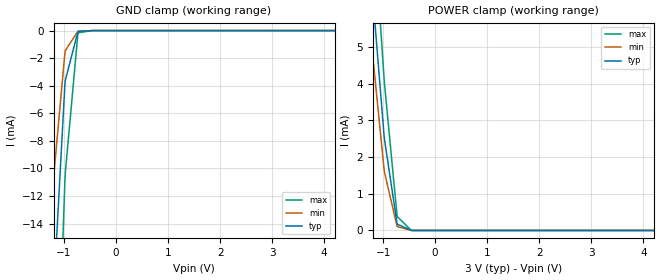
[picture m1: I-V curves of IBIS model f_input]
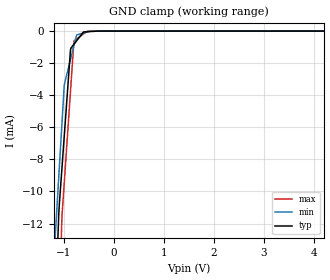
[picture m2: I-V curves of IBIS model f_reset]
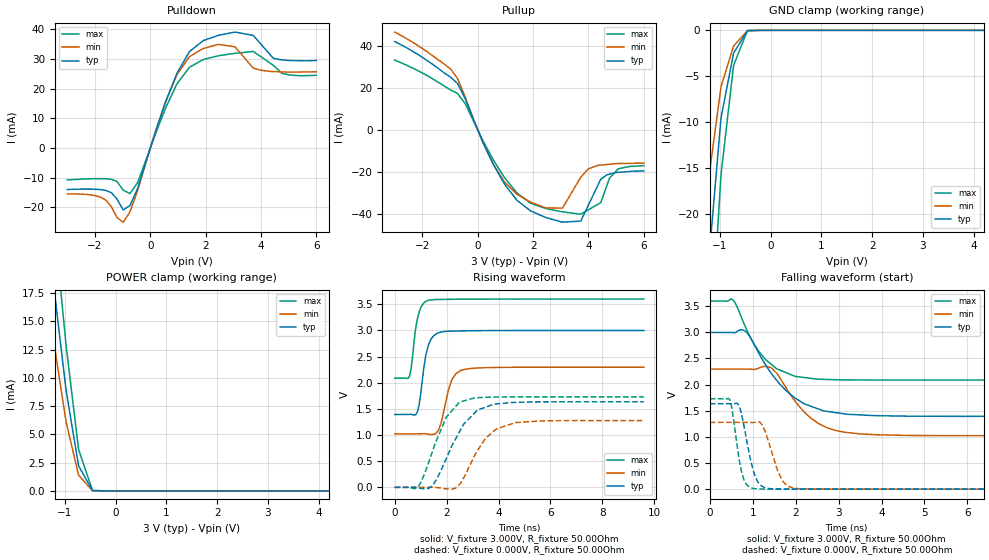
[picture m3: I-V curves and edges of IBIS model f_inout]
[IBIS Ver]   3.2
[File Name]   rc_p33_30v_128m_b.ibs
[File Rev]   1.01
[Date]   8/21/2009
[Source]   From silicon level SPICE model at Numonyx B.V.
[Notes]   The following information corresponds to the
   Redcliff 65nm P33 128Mb chip with EZBGA package.
[Disclaimer]   This information is for modeling purposes only and is not
   guaranteed.Numonyx B.V. is not responsible for any problem
   this model may cause to customers.
[Copyright]   Copyright 2009, Numonyx B.V., All Rights Reserved.
[Component]   P33_30V_128M_EZBGA
[Manufacturer]  Numonyx B.V.
[Package]
|   typ   min   max
R_pkg   0.33Ohm   0.16Ohm   0.50Ohm
L_pkg   6.77nH   3.42nH   10.12nH
C_pkg   1.25pF   0.27pF   2.23pF
[PIN]   signal_name   model_name   R_pin   L_pin   C_pin
A1   A0   f_input   0.28   5.77nH   0.65pF
A2   A5   f_input   0.36   7.41nH   0.92pF
A3   A7   f_input   0.20   4.23nH   0.40pF
A4   NC   NC
A5   A12   f_input   0.16   3.42nH   0.27pF
A6   VCC   POWER
A7   A17   f_input   0.26   5.74nH   0.67pF
A8   A21   f_input   0.33   7.38nH   0.83pF
B1   A1   f_input   0.27   5.51nH   0.60pF
B2   VSS   GND
B3   A8   f_input   0.35   7.25nH   0.89pF
B4   CE#   f_input   0.43   8.13nH   1.28pF
B5   A13   f_input   0.23   4.66nH   0.46pF
B6   NC   NC
B7   A18   f_input   0.26   5.62nH   0.64pF
B8   NC   NC
C1   A2   f_input   0.29   5.77nH   0.64pF
C2   A6   f_input   0.29   5.73nH   0.64pF
C3   A9   f_input   0.35   7.03nH   0.85pF
C4   A11   f_input   0.34   6.86nH   0.82pF
C5   A14   f_input   0.27   5.44nH   0.59pF
C6   WP#   f_input   0.27   5.44nH   0.59pF
C7   A19   f_input   0.41   8.27nH   1.06pF
C8   A20   f_input   0.33   6.76nH   0.81pF
D1   A3   f_input   0.30   6.07nH   0.69pF
D2   A4   f_input   0.28   5.47nH   0.59pF
D3   A10   f_input   0.37   7.50nH   0.93pF
D4   RST#   f_reset   0.32   6.25nH   0.83pF
D5   VCCQ   POWER
D6   VCCQ   POWER
D7   A15   f_input   0.25   4.83nH   0.48pF
D8   A16   f_input   0.29   5.71nH   0.62pF
E1   D8   f_inout   0.28   6.28nH   0.82pF
E2   D1   f_inout   0.26   5.20nH   0.63pF
E3   D9   f_inout   0.25   4.92nH   0.56pF
E4   D3   f_inout   0.25   4.98nH   0.58pF
E5   D4   f_inout   0.30   5.87nH   0.65pF
E6   CLK   f_input   0.29   5.72nH   0.73pF
E7   D15   f_inout   0.27   5.36nH   0.56pF
E8   NC   NC
F1   NC   NC
F2   D0   f_inout   0.21   4.33nH   0.46pF
F3   D10   f_inout   0.23   4.69nH   0.55pF
F4   D11   f_inout   0.23   4.60nH   0.52pF
F5   D12   f_inout   0.20   4.02nH   0.43pF
F6   ADV#   f_input   0.25   4.85nH   0.49pF
F7   WAIT   f_inout   0.24   4.71nH   0.53pF
F8   OE#   f_input   0.42   9.70nH   2.23pF
G1   A22   f_input   0.47   10.12nH   1.28pF
G2   NC   NC
G3   D2   f_inout   0.22   4.43nH   0.42pF
G4   VCCQ   POWER
G5   D5   f_inout   0.17   3.51nH   0.35pF
G6   D6   f_inout   0.18   3.76nH   0.40pF
G7   D14   f_inout   0.22   4.44nH   0.42pF
G8   WE#   f_input   0.50   9.96nH   1.33pF
H1   NC   NC
H2   VSSQ   GND
H3   VCC   POWER
H4   VSS   GND
H5   D13   f_inout   0.21   4.31nH   0.41pF
H6   VSSQ   GND
H7   D7   f_inout   0.23   4.67nH   0.46pF
H8   NC   NC
| Models and submodels in the file (3): f_input (Input), f_reset (Input), f_inout (I/O)
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[Model]   f_input
Model_type   Input
Vinl = 0.400V
Vinh = 2.600V
|   typ   min   max
C_comp   6.000pF   2.000pF   7.000pF
[Voltage Range]   3.000V   2.300V   3.600V
[Temperature Range]   25.0   85.0   -40.0
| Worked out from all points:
|   GND clamp passes 1 mA (typ) near -0.79 V on its own axis
|   POWER clamp passes 1 mA (typ) near -0.82 V on its own axis
[GND Clamp]
|   Voltage   I(typ)   I(min)   I(max)
-3V       -214.2mA   -171.1mA   -282mA
-1.398V   -38.01mA   -24.9mA    -60.4mA
-1.209V   -20.02mA   -11.33mA   -36.27mA
-1.2V     -19.19mA   -10.72mA   -35.15mA
-984mV    -4.085mA   -1.721mA   -11.16mA
-975mV    -3.631mA   -1.46mA    -10.38mA
-732mV    -88.55uA   -49.57uA   -226.8uA
-723mV    -64.96uA   -39.8uA    -159.9uA
-453mV    -377.4nA   -554.6nA   -216.8nA
6V        0A         0A         0A
[POWER Clamp]
|   Voltage   I(typ)   I(min)   I(max)
-3V       44.58mA    39.22mA    51.64mA
-1.299V   8.339mA    6.46mA     11.02mA
-1.209V   6.572mA    4.919mA    8.979mA
-1.2V     6.398mA    4.769mA    8.776mA
-984mV    2.624mA    1.697mA    4.188mA
-975mV    2.493mA    1.595mA    4.017mA
-732mV    187.3uA    115.4uA    401uA
-723mV    168.4uA    103.4uA    368.4uA
-453mV    1.105uA    1.525uA    700.3nA
6V        0A         0A         0A
[Model]   f_reset
Model_type   Input
Vinl = 0.400V
Vinh = 2.600V
|   typ   min   max
C_comp   6.000pF   2.000pF   7.000pF
[Voltage Range]   3.000V   2.300V   3.600V
[Temperature Range]   25.0   85.0   -40.0
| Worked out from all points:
|   GND clamp passes 1 mA (typ) near -0.84 V on its own axis
[GND Clamp]
|   Voltage   I(typ)   I(min)   I(max)
-3V       -205.4mA   -173mA     -256.3mA
-1.209V   -20.5mA    -14.72mA   -29.6mA
-1.101V   -11.42mA   -9.082mA   -18.23mA
-1.047V   -8.959mA   -6.264mA   -12.54mA
-1.038V   -8.571mA   -5.795mA   -11.6mA
-993mV    -6.627mA   -3.447mA   -9.54mA
-867mV    -1.187mA   -1.777mA   -3.783mA
-795mV    -811.6uA   -873.4uA   -609.4uA
-741mV    -594.7uA   -238.1uA   -486.6uA
-606mV    -54.38uA   -121.6uA   -179.4uA
-318mV    -41.02nA   -2.805uA   -2.579uA
6V        0A         0A         0A
[POWER Clamp]
|   Voltage   I(typ)   I(min)   I(max)
-3V       0A         0A         0A
0V        0A         0A         0A
2.301V    0A         0A         0A
3.003V    0A         0A         0A
3.597V    0A         0A         0A
6V        0A         0A         0A
|Note: Typical Pullup/Pulldown I-V drives the most current due to
|silicon process output compensation setting.
[Model]   f_inout
Model_type   I/O
Vinl = 0.400V
Vinh = 2.600V
Vmeas = 1.500V
Vref = 1.500V
Cref = 30.0pF
|   typ   min   max
C_comp   4.000pF   2.000pF   5.000pF
[Voltage Range]   3.000V   2.300V   3.600V
[Temperature Range]   25.0   85.0   -40.0
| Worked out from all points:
|   slope of the pulldown table from 0 to 0.45 V, typ, clamps not added: 35.3 ohm
|   slope of the pullup table from 0 to 0.45 V, typ, clamps not added: 33.6 ohm
|   falling waveform, V_fixture 3.000V, R_fixture 50.00Ohm: 20-80 % time 950ps typ, 795ps min, 698ps max; typ from 3 V to 1.39 V
|   rising waveform, V_fixture 3.000V, R_fixture 50.00Ohm: 20-80 % time 294ps typ, 376ps min, 254ps max; typ from 1.39 V to 3 V
|   rising waveform, V_fixture 0.000V, R_fixture 50.00Ohm: 20-80 % time 1.07ns typ, 959ps min, 850ps max; typ from 0.001 V to 1.64 V
|   falling waveform, V_fixture 0.000V, R_fixture 50.00Ohm: 20-80 % time 252ps typ, 311ps min, 193ps max; typ from 1.64 V to 0.001 V
[Pulldown]
|   Voltage   I(typ)   I(min)   I(max)
-3V       -13.95mA   -15.43mA   -10.69mA
-1.749V   -14.03mA   -16.72mA   -10.29mA
-975mV    -20.83mA   -24.95mA   -14.15mA
-732mV    -19.35mA   -21.46mA   -15.33mA
-453mV    -13.45mA   -14.2mA    -11.51mA
186mV     5.442mA    5.555mA    4.728mA
960mV     25.11mA    24.64mA    21.55mA
1.914V    36.21mA    33.56mA    29.84mA
3.057V    39.08mA    34.14mA    31.92mA
3.723V    37.95mA    26.93mA    32.57mA
4.452V    30.24mA    25.78mA    27.85mA
6V        29.52mA    25.73mA    24.53mA
[GND Clamp]
|   Voltage   I(typ)   I(min)   I(max)
-3V       -196.6mA   -150.6mA   -237mA
-1.398V   -40.49mA   -27.36mA   -56.22mA
-1.209V   -24.51mA   -15.77mA   -36.56mA
-1.2V     -23.78mA   -15.24mA   -35.64mA
-984mV    -9.872mA   -6.357mA   -16.19mA
-975mV    -9.406mA   -6.06mA    -15.51mA
-732mV    -2.522mA   -1.731mA   -3.878mA
-453mV    -32.92uA   -41.65uA   -18.68uA
6V        0A         0A         0A
[Pullup]
|   Voltage   I(typ)   I(min)   I(max)
-3V       42.3mA     46.8mA     33.41mA
-1.2V     27.2mA     31.42mA    20.94mA
-732mV    22.27mA    24.61mA    17.46mA
555mV     -16.23mA   -16.15mA   -14.11mA
1.41V     -33.49mA   -30.61mA   -29.96mA
1.914V    -38.68mA   -34.5mA    -35mA
3.057V    -44.01mA   -37.29mA   -39.05mA
3.723V    -43.46mA   -22.52mA   -40.21mA
4.452V    -23.42mA   -16.75mA   -34.44mA
4.758V    -21.09mA   -16.36mA   -23.08mA
5.073V    -20.21mA   -16mA      -18.57mA
6V        -19.56mA   -15.84mA   -17.03mA
[POWER Clamp]
|   Voltage   I(typ)   I(min)   I(max)
-3V       101.9mA    81.99mA    120.9mA
-1.389V   25.34mA    19.02mA    32.68mA
-1.281V   20.78mA    15.37mA    27.29mA
-1.2V     17.37mA    12.65mA    23.25mA
-1.191V   17.03mA    12.38mA    22.83mA
-984mV    9.151mA    6.303mA    13.18mA
-975mV    8.843mA    6.071mA    12.79mA
-732mV    2.254mA    1.421mA    3.717mA
-453mV    29.5uA     19.11uA    45.13uA
6V        0A         0A         0A
[Ramp]
R_load = 50.00Ohm
|   typ   min   max
dV/dt_r   980.615mV/1.067ns   765.325mV/958.643ps   1.037V/849.772ps
dV/dt_f   962.719mV/949.930ps 764.159mV/794.496ps 906.432mV/698.117ps
[Falling Waveform]
V_fixture = 3.000V
V_fixture_min = 2.300V
V_fixture_max = 3.600V
R_fixture = 50.00Ohm
|   Time   V(typ)   V(min)   V(max)
0s        2.998V     2.297V     3.599V
520ps     2.997V     2.297V     3.632V
630ps     3.013V     2.297V     3.502V
830ps     3.02V      2.297V     3.105V
1.14ns    2.604V     2.316V     2.638V
1.43ns    2.218V     2.323V     2.39V
1.99ns    1.741V     1.68V      2.158V
2.55ns    1.528V     1.247V     2.103V
3.49ns    1.421V     1.058V     2.089V
9.6ns     1.393V     1.023V     2.088V
[Rising Waveform]
V_fixture = 3.000V
V_fixture_min = 2.300V
V_fixture_max = 3.600V
R_fixture = 50.00Ohm
|   Time   V(typ)   V(min)   V(max)
0s        1.393V     1.023V     2.088V
570ps     1.395V     1.023V     2.125V
880ps     1.451V     1.023V     3.233V
1.04ns    1.951V     1.026V     3.468V
1.2ns     2.532V     1.024V     3.552V
1.29ns    2.712V     1.017V     3.576V
1.69ns    2.953V     1.095V     3.591V
2.19ns    2.986V     2.044V     3.594V
2.55ns    2.99V      2.235V     3.597V
9.6ns     2.998V     2.297V     3.599V
[Rising Waveform]
V_fixture = 0.000V
V_fixture_min = 0.000V
V_fixture_max = 0.000V
R_fixture = 50.00Ohm
|   Time   V(typ)   V(min)   V(max)
0s        923.1uV    1.776mV    585.5uV
860ps     -4.502mV   1.636mV    -8.437mV
1.04ns    -20.53mV   1.544mV    134mV
1.4ns     9.133mV    2.684mV    610.2mV
1.99ns    555.7mV    -27.13mV   1.343V
2.5ns     1.067V     60.03mV    1.63V
3.19ns    1.479V     703.9mV    1.714V
3.91ns    1.595V     1.115V     1.728V
5.69ns    1.634V     1.272V     1.729V
9.6ns     1.635V     1.277V     1.729V
[Falling Waveform]
V_fixture = 0.000V
V_fixture_min = 0.000V
V_fixture_max = 0.000V
R_fixture = 50.00Ohm
|   Time   V(typ)   V(min)   V(max)
0s        1.635V     1.277V     1.729V
470ps     1.635V     1.277V     1.7V
650ps     1.637V     1.277V     759.9mV
750ps     1.394V     1.277V     299.1mV
960ps     528.1mV    1.275V     23.6mV
1.07ns    220.6mV    1.284V     8.797mV
1.2ns     62.79mV    1.25V      3.749mV
1.68ns    3.562mV    178.3mV    1.252mV
1.94ns    2.501mV    20.54mV    833.8uV
9.6ns     923.1uV    1.776mV    585.5uV
